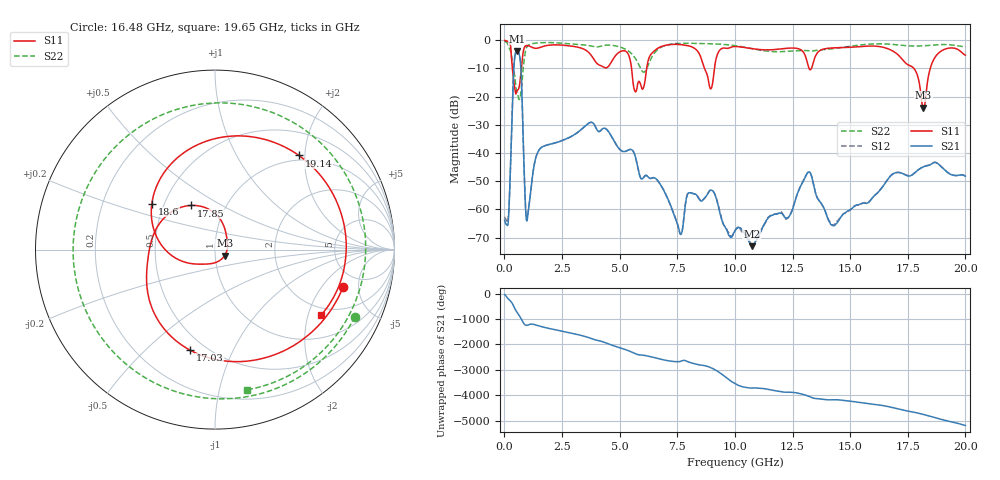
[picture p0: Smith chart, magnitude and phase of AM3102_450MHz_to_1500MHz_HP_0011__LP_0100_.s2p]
!Agilent Technologies,E8364B,MY43040894,A.07.50.67
!Agilent E8364B: A.07.50.67
!Date: Thursday, January 11, 2018 05:31:06
!Correction: S11(Full 2 Port(1,2))
!S21(Full 2 Port(1,2))
!S12(Full 2 Port(1,2))
!S22(Full 2 Port(1,2))
!S2P File: Measurements: S11, S21, S12, S22:
# Hz S  dB  R 50
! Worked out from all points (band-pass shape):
!   1601 points, 10 MHz to 20 GHz, reference 50 ohm
!   highest |S21| = -3.76 dB at 547.2 MHz (marker M1); lowest = -73.1 dB at 10.73 GHz (marker M2)
!   |S21| within 3 dB of the highest: 439.4 MHz to 683.6 MHz (244.2 MHz wide, 43.5 % of centre)
!   lowest |S11| = -23.9 dB at 18.18 GHz (marker M3), VSWR 1.14, Z = 55.6 - j3.74 ohm
!   |S11| at or under -10 dB: 5.518 GHz to 6.172 GHz (654.2 MHz wide, 11.2 % of centre); 8.683 GHz to 9.111 GHz (428 MHz wide, 4.81 % of centre); 17.77 GHz to 18.47 GHz (705.9 MHz wide, 3.9 % of centre)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
!   |S22| runs from -21.0 to -0.3 dB; largest |S21 - S12| = 0.0017
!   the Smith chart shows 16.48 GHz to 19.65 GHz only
!   S11 on the Smith chart (normalised r, x): 16.48 GHz: 3.58, -3.33; 17.03 GHz: 0.41, -0.69; 17.85 GHz: 0.69, +0.37; 18.6 GHz: 0.43, +0.27; 19.14 GHz: 0.91, +1.88; 19.65 GHz: 1.73, -2.43
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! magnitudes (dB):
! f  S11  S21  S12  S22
! 10 MHz  -0.1  -63.8  -62.6  -0.3
! 547.2 MHz  -18.1  -3.8  -3.8  -18.3
! 997 MHz  -1.9  -63.3  -63.1  -2.1
! 1.509 GHz  -2.6  -38.9  -38.9  -0.9
! 3.346 GHz  -2.8  -31.6  -31.6  -1.6
! 5.695 GHz  -18.3  -41.7  -41.7  -6.6
! 6.682 GHz  -2.7  -50.1  -50.2  -3.1
! 7.631 GHz  -1.5  -68.8  -68.9  -1.1
! 8.956 GHz  -17.2  -53.2  -53.1  -1.2
! 10.01 GHz  -2.2  -67.7  -67.6  -1.9
! 10.73 GHz  -2.9  -73.1  -72.5  -3.0
! 13.34 GHz  -9.6  -48.6  -48.6  -3.8
! 14.25 GHz  -2.7  -65.7  -65.5  -3.0
! 16.48 GHz  -2.6  -51.2  -51.2  -1.3
! 16.68 GHz  -3.1  -48.8  -48.8  -1.4
! 17.03 GHz  -4.8  -46.9  -46.9  -1.6
! 17.85 GHz  -11.1  -46.7  -46.7  -2.0
! 18.18 GHz  -23.9  -44.9  -44.9  -2.0
! 18.6 GHz  -7.2  -43.5  -43.5  -1.7
! 19.14 GHz  -3.1  -46.3  -46.3  -1.5
! 19.65 GHz  -3.2  -47.9  -48.0  -1.9
! 20 GHz  -5.3  -48.2  -48.1  -2.3
